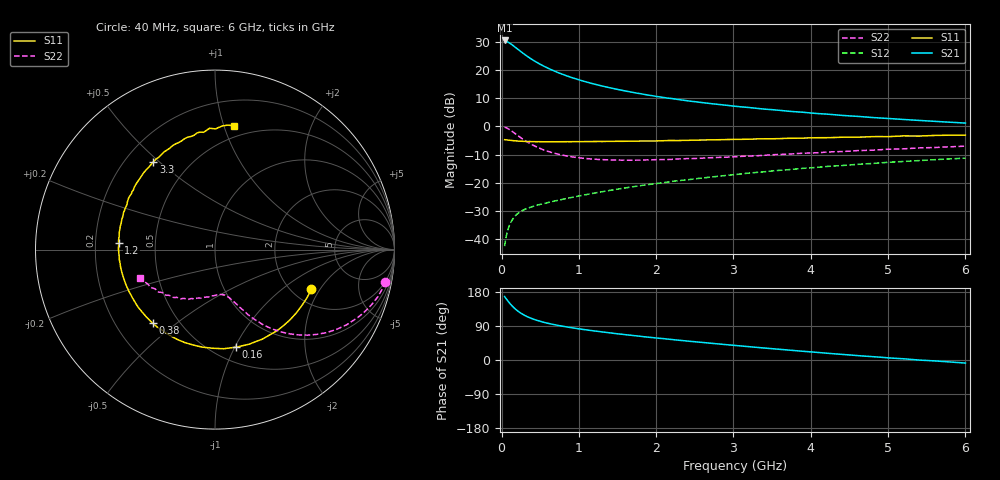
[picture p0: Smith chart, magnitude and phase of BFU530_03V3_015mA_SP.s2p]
! Filename:  P:\Prog\Test\Noise\ATS_data\Testdata_Net\03 Spar\BFU530_APG2013_40_A05_03p3V_015mA_SP_CM01_D.s2p
! Date/Time: Fri 26/Apr/2013 13:03:16
! BFU530_APG2013_40_A05_03p3V_1to25mA_SP_CM01_Bias6_R.s2p
! MDIF S-parameter v. bias file
! BFU530_APG2013_40_A05_03p3V_1to25mA_SP_CM01
! Date/time Wed Apr 24 18:17:07 2013
! VAR V_out= 3.3000
! VAR I_out= 14.9950
! VAR V_in= 0.8452
! VAR I_in= 0.1706
! Device data file deembeded for feedlines and parallel
! Original file: \03 Spar\BFU530_APG2013_40_A05_03p3V_015mA_SP_CM01_R.s2p
! Feed-files: PR047V01_250413_Feed1.s2p, PR047V01_250413_Feed2.s2p
! Parallel-file: PR047V01_250413_Par.s2p
# MHz S MA R 50
!  Freq-MHz  S11-mag  S11-arg  S21-mag  S21-arg  S12-mag  S12-arg  S22-mag  S22-arg
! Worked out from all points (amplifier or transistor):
!   98 points, 40 MHz to 6 GHz, reference 50 ohm
!   highest |S21| = 30.4 dB at 40 MHz (marker M1)
!   |S21| within 3 dB of that: start of sweep to 205.3 MHz
!   unconditionally stable (mu >= 1): 1.404 GHz to 3.743 GHz
!   at 300 MHz: K = 0.41, MSG = 27.4 dB, |S12| = -29.4 dB
!   at 1.6 GHz: K = 1.03, MAG = 16.1 dB, |S12| = -21.8 dB
!   at 6 GHz: K = 0.86, MSG = 6.2 dB, |S12| = -11.3 dB
!   S11 on the Smith chart (normalised r, x): 40 MHz: 2.52, -1.68; 160 MHz: 0.64, -1.01; 380 MHz: 0.36, -0.41; 1.2 GHz: 0.30, +0.03; 3.3 GHz: 0.31, +0.48; 6 GHz: 0.40, +1.08
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40  0.5812 -22.4  33.23 167.6  0.007538 81.3  0.9661 -10.7
50  0.5784 -27.9  33.01 164.1  0.009335 79.1  0.9571 -13.3
80  0.5723 -43.3  31.28 156.3  0.01432 72.9  0.9146 -20.9
100  0.5686 -52.9  30.09 151.3  0.01725 69.2  0.8807 -25.4
120  0.5643 -62.1  28.92 146.4  0.01989 66.0  0.8451 -29.7
160  0.5562 -78.0  26.27 138.0  0.02433 60.6  0.7729 -36.8
200  0.5498 -91.5  23.82 131.0  0.02779 56.5  0.7027 -42.7
260  0.5445 -107.9  20.61 122.4  0.03171 52.6  0.6141 -49.4
320  0.5397 -120.4  17.95 115.7  0.0347 50.1  0.543 -54.3
380  0.537 -130.3  15.76 110.3  0.03712 48.8  0.486 -58.0
480  0.5349 -142.7  13.04 103.4  0.04077 48.1  0.4166 -62.4
600  0.5328 -153.8  10.75 96.9  0.04468 48.6  0.3609 -65.9
800  0.5342 -166.6  8.248 88.8  0.05136 50.3  0.3069 -70.3
1050  0.5365 -178.6  6.377 80.8  0.06008 52.4  0.2732 -74.8
1200  0.5386 175.8  5.604 76.6  0.0656 53.3  0.2623 -77.3
1600  0.5443 163.1  4.231 66.8  0.081 54.6  0.2522 -84.1
2050  0.5539 152.1  3.314 57.2  0.09871 54.5  0.2572 -92.3
3100  0.5889 128.9  2.216 37.0  0.1435 51.2  0.2939 -111.5
3300  0.5982 125.0  2.085 33.3  0.1526 50.1  0.3013 -115.1
4100  0.6289 110.3  1.681 19.8  0.1886 44.8  0.3413 -128.8
5200  0.6769 92.5  1.324 3.2  0.2389 36.1  0.3993 -146.9
6000  0.697 81.2  1.143 -8.1  0.2736 28.7  0.4462 -159.4
